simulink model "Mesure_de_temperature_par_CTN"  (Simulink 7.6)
settings: Solver=ode23t  StartTime=0.0  StopTime=10  RelTol=1e-3
InitFcn:
  | clc, delete *.mat
StopFcn:
  | % lecture du fichier binaire
  | load thermistance.mat
  | 
  | % trace de la tension et du courant d’induit
  | plotyy(x(1,:),x(2,:),x(1,:),x(3,:))
  | title('Résistance de la thermistance')
  | grid
libraries: nesl_utility x3, MaLibrairieElectrical_lib x1

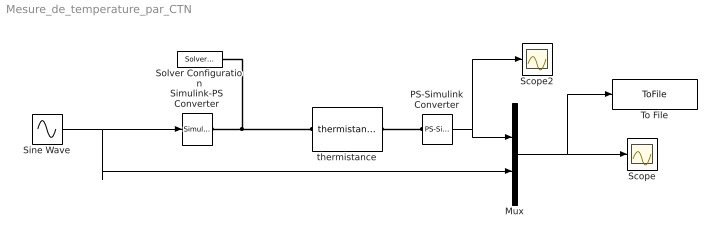
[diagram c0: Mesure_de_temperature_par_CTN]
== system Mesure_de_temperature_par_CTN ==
  Mux : Mux  Inputs=2
  PS-Simulink Converter : nesl_utility/PS-Simulink Converter  DialogController=NetworkEngine.DynNeUtilDlgSource  SystemSampleTime=-1  PhysicalDomain=network_engine_domain  LeftPortType=input  RightPortType=output  SubClassName=ps_output  Unit=1  AffineConversion=off
  Scope : Scope
  Scope2 : Scope
  Simulink-PS Converter : nesl_utility/Simulink-PS Converter  DialogController=NetworkEngine.DynNeUtilDlgSource  SystemSampleTime=-1  PhysicalDomain=network_engine_domain  LeftPortType=input  RightPortType=output  SubClassName=ps_input  Unit=1  AffineConversion=off  InputFilterTimeConstant=.001  UdotUserProvided=0
  Sine Wave : Sin  Amplitude=100  Bias=300  SampleTime=0
  Solver Configuration : nesl_utility/Solver Configuration  DialogController=NetworkEngine.DynNeUtilDlgSource  SystemSampleTime=-1  PhysicalDomain=network_engine_domain  LeftPortType=input  RightPortType=generic  SubClassName=solver  Accelerate=off  Profile=off  ResidualTolerance=1e-9  MaxNonlinIter=3  MaxModeIter=2  DoFixedCost=off  UseLocalSampling=off  DoDC=off  LinearAlgebra=Sparse  LocalSolverSampleTime=.001  LocalSolverChoice=NE_BACKWARD_EULER_ADVANCER  UseLocalSolver=off
  To File : ToFile  Filename=thermistance  MatrixName=x
  thermistance : MaLibrairieElectrical_lib/thermistance  DialogController=NetworkEngine.DynNeDlgSource  SystemSampleTime=-1  T0=300 K  B=2.9e+3 K  R0=100 Ohm  LocalVarLogging=[]
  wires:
  PS-Simulink Converter/1 -> Mux/1, Scope2/1
  Mux/1 -> Scope/1, To File/1
  Sine Wave/1 -> Simulink-PS Converter/1, Mux/2
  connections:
  Simulink-PS Converter/RConn1 -- thermistance/LConn1 -- Solver Configuration/RConn1
  thermistance/RConn1 -- PS-Simulink Converter/LConn1
